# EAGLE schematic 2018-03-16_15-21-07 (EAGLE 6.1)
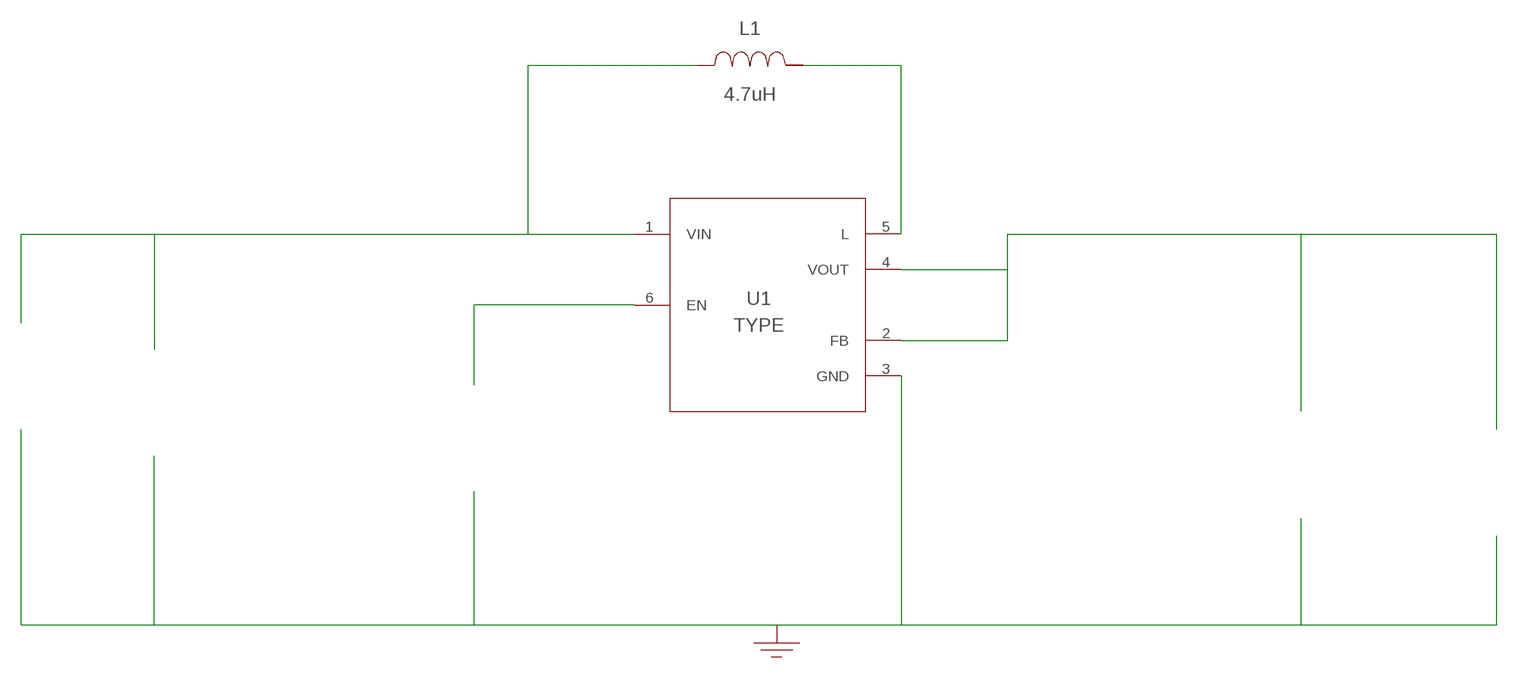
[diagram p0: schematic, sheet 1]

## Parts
CIN  10uF  GRM21BR60J106ME19LGRM21BR60J106ME19L  [0805]  (not placed on a sheet)
COUT  10uF  C0805C106K8PACTUC0805C106K8PACTU  [0805]  (not placed on a sheet)
GND  WB_GND  WB_GNDWB_GND  [WB_GND]
IOUT  WB_CURRENT_LOAD  WB_CURRENT_LOADWB_CURRENT_LOAD  [WB_CURRENT_LOAD]  (not placed on a sheet)
L1  4.7uH  LQM2HPN4R7MGCLLQM2HPN4R7MGCL  [1008]
U1  TPS61222DCKR  TPS61222DCKRTPS61222DCKR  [DCK0006A]
VEN  WB_PRIM_DC_VOLTAGE_SOURCE  WB_PRIM_DC_VOLTAGE_SOURCEWB_PRIM_DC_VOLTAGE_SOURCE  [WB_PRIM_DC_VOLTAGE_SOURCE]  (not placed on a sheet)
VIN  WB_BATTERY  WB_BATTERYWB_BATTERY  [WB_BATTERY]  (not placed on a sheet)

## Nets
0: Cin.2@2 Cout.2@2 GND.1 Iout.-@2 U1.3(GND) Ven.-@2 Vin.-@2
1: U1.6(EN) Ven.+@1
2: Cin.1@1 L1.1 U1.1(VIN) Vin.+@1
3: Cout.1@1 Iout.+@1 U1.2(FB) U1.4(VOUT)
4: L1.2 U1.5(L)
Unconnected: CIN.1 CIN.2 COUT.1 COUT.2 IOUT.1(+) IOUT.2(-) VEN.1(+) VEN.2(-) VIN.1(+) VIN.2(-)

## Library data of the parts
CIN = AcceleratedDesigns_Lib:GRM21BR60J106ME19L; Cap: 1.0E-5; ESR: 0.0030; IRMS: 0.0; Manufacturer_Name: MuRata; Manufacturer_Part_Number: GRM21BR60J106ME19L; VDC: 6.3; Vendor: MuRata
COUT = AcceleratedDesigns_Lib:C0805C106K8PACTU; Cap: 1.0E-5; ESR: 0.0030; IRMS: 11.43; Manufacturer_Name: Kemet; Manufacturer_Part_Number: C0805C106K8PACTU; VDC: 10.0; Vendor: Kemet
GND = AcceleratedDesigns_Lib:WB_GND; Manufacturer_Name: WB_GND; Manufacturer_Part_Number: WB_GND; PowerPortType: POWER_GROUND; Value: Value
IOUT = AcceleratedDesigns_Lib:WB_CURRENT_LOAD; Manufacturer_Name: WB_CURRENT_LOAD; Manufacturer_Part_Number: WB_CURRENT_LOAD; PowerPortType: POWER_GROUND; Value: Value
L1 = AcceleratedDesigns_Lib:LQM2HPN4R7MGCL; DCR: 0.18; IDC: 0.8; L: 4.7E-6; Manufacturer_Name: MuRata; Manufacturer_Part_Number: LQM2HPN4R7MGCL; Vendor: MuRata
U1 = AcceleratedDesigns_Lib:TPS61222DCKR; CompType: IC; Manufacturer: Texas Instruments; Manufacturer_Name: Texas Instruments; Manufacturer_Part_Number: TPS61222DCKR; MountType: SMT; PIN_COUNT: 6; PackageReference: DCK0006A; PartNumber: TPS61222DCK; RefDes: RefDes; RoHS: Y; TYPE: TYPE; Value: Value
VEN = AcceleratedDesigns_Lib:WB_PRIM_DC_VOLTAGE_SOURCE; Manufacturer_Name: WB_PRIM_DC_VOLTAGE_SOURCE; Manufacturer_Part_Number: WB_PRIM_DC_VOLTAGE_SOURCE; PowerPortType: POWER_GROUND; Value: Value
VIN = AcceleratedDesigns_Lib:WB_BATTERY; Manufacturer_Name: WB_BATTERY; Manufacturer_Part_Number: WB_BATTERY; PowerPortType: POWER_GROUND; Value: Value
